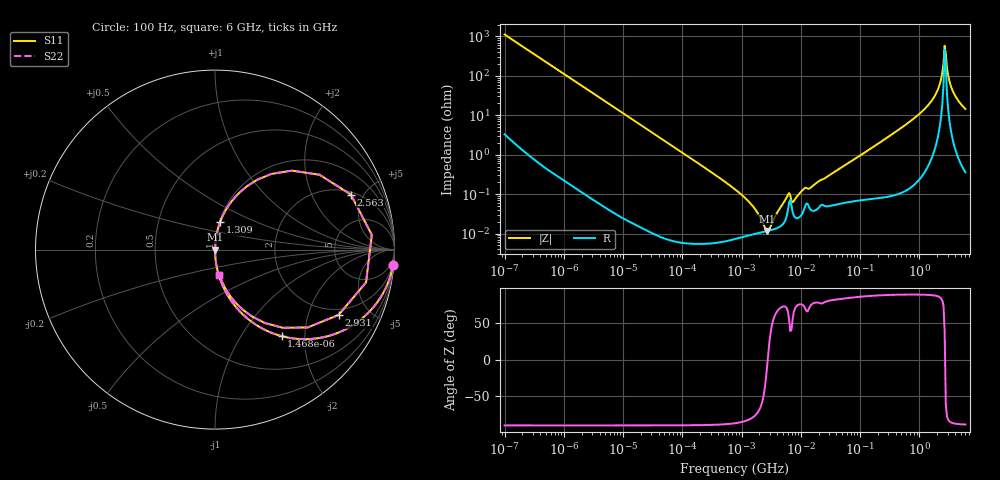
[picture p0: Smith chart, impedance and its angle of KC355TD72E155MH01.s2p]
!Murata Part Number: KC355TD72E155MH01
!These Parameters are Measured in Series Mode Connection
!Data Generated on Mar 13, 2026
!  o--ll--o
!Port1  Port2
!  o------o
!Operation Temp=25[degC], DC Bias Voltage=0[V]
!Freq. Start=100[Hz] Stop=6[GHz] 401[Steps]
# Hz S RI R 50
!Freq.(Hz) S11(Real) S11(Imag) S21(Real) S21(Imag) S12(Real) S12(Imag) S22(Real) S22(Imag)
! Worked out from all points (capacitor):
!   401 points, 100 Hz to 6 GHz, reference 50 ohm
!   read as one part in series: C = 1.42 uF near 109 Hz
!   lowest |Z| = 11.7 mohm at 2.714 MHz (marker M1)
!   series resonance near 2.762 MHz, so ESL is about 2.3 nH
!   S11 on the Smith chart (normalised r, x): 100 Hz: 1, -22; 1.468 kHz: 1.00, -1.53; 1.309 GHz: 1.01, +0.32; 2.563 GHz: 2.18, +4.01; 2.931 GHz: 1.72, -3.18; 6 GHz: 1.01, -0.29
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100  0.9919 -0.0884  0.00813 0.0884  0.00813 0.0884  0.9919 -0.0884
438  0.8676 -0.3379  0.1324 0.3379  0.1324 0.3379  0.8676 -0.3379
1468  0.3707 -0.482  0.6293 0.482  0.6293 0.482  0.3707 -0.482
2008  0.2398 -0.4259  0.7602 0.4259  0.7602 0.4259  0.2398 -0.4259
5378  0.0425 -0.2007  0.9575 0.2007  0.9575 0.2007  0.0425 -0.2007
40335  0.00087 -0.028  0.9991 0.028  0.9991 0.028  0.00087 -0.028
774597  7.45e-05 -0.00132  0.9999 0.00132  0.9999 0.00132  7.45e-05 -0.00132
1585629  9.67e-05 -0.000464  0.9999 0.000464  0.9999 0.000464  9.67e-05 -0.000464
2713602  0.000116 -1.38e-05  0.9999 1.38e-05  0.9999 1.38e-05  0.000116 -1.38e-05
6075234  0.000405 0.000875  0.9996 -0.000875  0.9996 -0.000875  0.000405 0.000875
7599586  0.000289 0.000604  0.9997 -0.000604  0.9997 -0.000604  0.000289 0.000604
1.137099e7  0.000413 0.00132  0.9996 -0.00132  0.9996 -0.00132  0.000413 0.00132
1.555665e7  0.000382 0.00153  0.9996 -0.00153  0.9996 -0.00153  0.000382 0.00153
3.124326e8  0.00175 0.0296  0.9982 -0.0296  0.9982 -0.0296  0.00175 0.0296
1.309207e9  0.0286 0.1542  0.9714 -0.1542  0.9714 -0.1542  0.0286 0.1542
1.95892e9  0.1397 0.3209  0.8603 -0.3209  0.8603 -0.3209  0.1397 0.3209
2.34314e9  0.4279 0.4401  0.5721 -0.4401  0.5721 -0.4401  0.4279 0.4401
2.562649e9  0.7573 0.3063  0.2427 -0.3063  0.2427 -0.3063  0.7573 0.3063
2.931063e9  0.689 -0.3638  0.311 0.3638  0.311 0.3638  0.689 -0.3638
3.205649e9  0.3779 -0.4357  0.6221 0.4357  0.6221 0.4357  0.3779 -0.4357
3.666503e9  0.1618 -0.3403  0.8382 0.3403  0.8382 0.3403  0.1618 -0.3403
6e9  0.0238 -0.1406  0.9762 0.1406  0.9762 0.1406  0.0238 -0.1406
